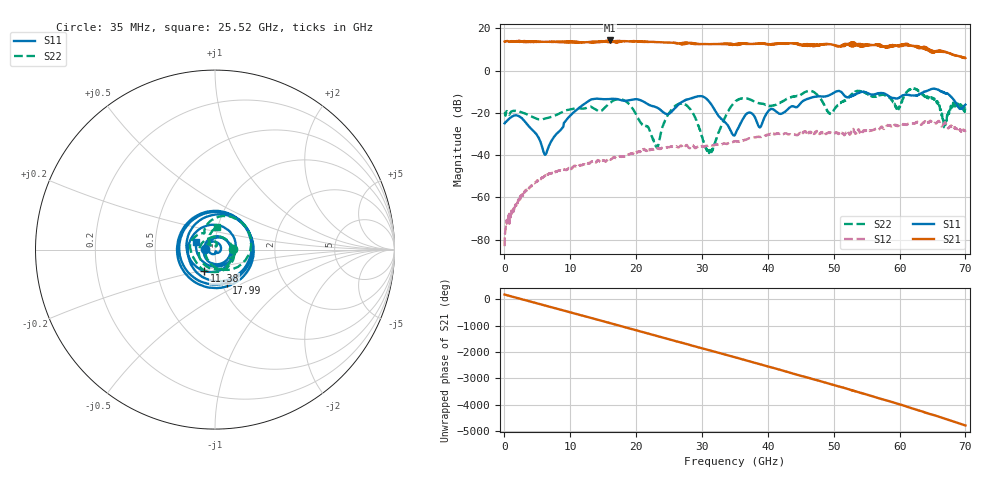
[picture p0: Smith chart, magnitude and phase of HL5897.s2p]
! 7/25/2023 10:50:37 AM
! H:\PROTOTYPE_DATA\65GHZ AMPLIFIER\PROTO1_CORRECTGD187PS.S2P
! CHANNEL.1
! TR.MEASUREMENT
! CORRECTED.DATA
# GHZ S RI R 50.0
! FREQ.GHZ  S11RE  S11IM  S21RE  S21IM  S12RE  S12IM  S22RE  S22IM
!; PortSelection: Port_12
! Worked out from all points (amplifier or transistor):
!   2000 points, 35 MHz to 70 GHz, reference 50 ohm
!   highest |S21| = 14.3 dB at 16.07 GHz (marker M1)
!   |S21| within 3 dB of that: start of sweep to 57.22 GHz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
!   unconditionally stable (mu >= 1): start of sweep to end of sweep
!   at 11.69 GHz: K = 17.87, MAG = 13.5 dB, |S12| = -44.8 dB
!   at 35.03 GHz: K = 5.49, MAG = 12.5 dB, |S12| = -33.4 dB
!   at 70 GHz: K = 6.37, MAG = 6.2 dB, |S12| = -28.4 dB
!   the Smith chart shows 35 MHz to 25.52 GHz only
!   S11 on the Smith chart (normalised r, x): 35 MHz: 0.89, +0.00; 11.38 GHz: 0.86, -0.21; 17.99 GHz: 1.06, -0.41; 25.52 GHz: 0.81, +0.07
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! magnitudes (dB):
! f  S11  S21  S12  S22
! 35 MHz  -24.9  13.8  -83.1  -20.2
! 2.45 GHz  -22.1  13.7  -59.5  -19.5
! 6.23 GHz  -39.7  13.7  -49.8  -22.6
! 11.38 GHz  -17.5  13.6  -44.9  -17.7
! 11.72 GHz  -16.6  13.3  -44.8  -17.9
! 16.07 GHz  -13.4  14.3  -42.0  -15.1
! 17.99 GHz  -14.1  13.9  -40.7  -13.8
! 23.38 GHz  -17.8  13.5  -36.6  -35.0
! 25.52 GHz  -19.0  13.3  -36.0  -18.0
! 28.11 GHz  -13.3  13.1  -36.7  -17.8
! 31.15 GHz  -14.8  12.6  -35.4  -38.1
! 35.03 GHz  -30.2  12.3  -33.4  -14.7
! 36.99 GHz  -19.9  12.7  -32.2  -13.3
! 38.81 GHz  -26.8  13.0  -31.4  -15.5
! 46.69 GHz  -12.7  12.4  -29.7  -9.7
! 49.49 GHz  -11.4  12.5  -29.4  -20.3
! 53.45 GHz  -11.0  12.3  -29.6  -9.6
! 58.34 GHz  -12.0  11.0  -25.9  -12.2
! 59.71 GHz  -13.1  11.8  -26.1  -18.4
! 62.48 GHz  -11.8  11.2  -24.7  -8.6
! 66.85 GHz  -10.6  9.0  -24.7  -24.6
! 70 GHz  -16.1  6.0  -28.4  -18.0
